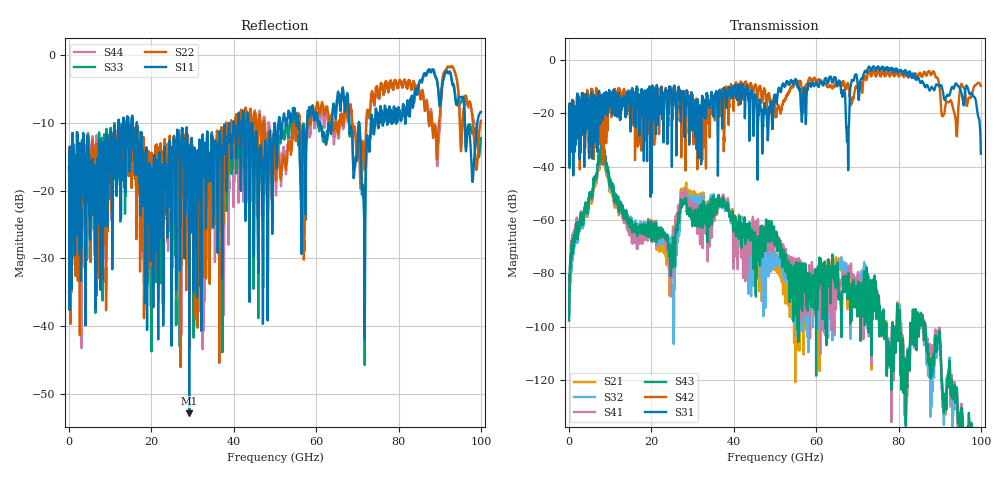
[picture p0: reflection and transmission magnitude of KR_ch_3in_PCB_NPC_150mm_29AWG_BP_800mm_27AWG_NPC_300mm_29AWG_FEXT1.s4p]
# GHz S RI R 45
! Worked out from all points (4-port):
!   4000 points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, 25 MHz to 100 GHz, reference 45 ohm
!   strongest paths, dB at 25 MHz, 25.02 GHz, 50.02 GHz, 75.03 GHz, 100 GHz:
!     S31: -21.2, -20.8, -13.2, -2.4, -35.2
!     S42: -21.3, -17.5, -18.0, -4.3, -9.8
!     S43: -97.6, -74.8, -66.5, -92.9, -139.2
!     S41: -94.8, -79.2, -67.1, -93.0, -140.7
!     S32: -94.7, -68.3, -75.2, -92.8, -145.1
!     S21: -88.7, -70.4, -77.9, -92.9, -145.9
!   lowest |S11| = -52.9 dB at 29.18 GHz (marker M1), VSWR 1.00, Z = 45.1 + j0.181 ohm
!   |S11| at or under -10 dB: start of sweep to 12.07 GHz; 16.48 GHz to 39.95 GHz (23.48 GHz wide, 83.2 % of centre); 44.4 GHz to 49.92 GHz (5.52 GHz wide, 11.7 % of centre)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
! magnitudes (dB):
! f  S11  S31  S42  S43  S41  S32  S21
! 25 MHz  -16.5  -21.2  -21.3  -97.6  -94.8  -94.7  -88.7
! 8 GHz  -15.1  -20.7  -25.9  -31.4  -33.0  -32.7  -34.4
! 24.02 GHz  -19.1  -22.2  -16.5  -68.5  -72.5  -68.8  -74.4
! 29.18 GHz  -52.9  -31.8  -16.4  -55.7  -52.9  -50.5  -48.9
! 67.6 GHz  -5.6  -27.9  -9.9  -87.9  -84.4  -81.9  -90.7
! 77.2 GHz  -9.6  -2.7  -4.6  -114.3  -114.7  -109.5  -112.3
! 100 GHz  -8.4  -35.2  -9.8  -139.2  -140.7  -145.1  -145.9
